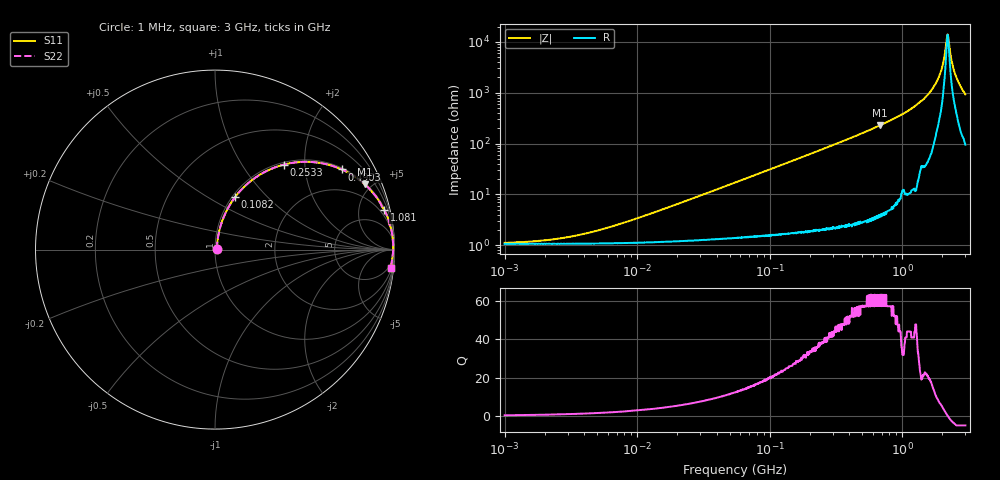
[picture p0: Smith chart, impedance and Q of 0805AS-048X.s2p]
!s-Parameter Generated by FASTRON Sdn. Bhd.
!FASTRON P/N : 0805AS-048X
!Keysight Technologies: E4991B_MY54100416_A.01.15
!Date: Mon Jun 15 12:50:52 2026
!Version  :Rev01  Mon Jun 15 12:50:52 2026
!Data & Calibration Information:
!Freq  S11  S21  S12  S22
!PortZ  Port1:50+j0  Port2:50+j0
!When reading reference impedance value at option line is always used.
! Remarks : This data is being provided solely for informational purposes.
# Hz S dB R 50
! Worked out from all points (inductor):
!   1601 points, 1 MHz to 3 GHz, reference 50 ohm
!   read as one part in series: L = 50.4 nH near 10.56 MHz
!   highest Q = 63.2 at 682.1 MHz (marker M1), where L = 53.2 nH
!   self-resonance near 2.2 GHz
!   S11 on the Smith chart (normalised r, x): 1 MHz: 1.02, +0.01; 108.2 MHz: 1.03, +0.67; 253.3 MHz: 1.04, +1.57; 490.3 MHz: 1.06, +3.13; 1.081 GHz: 1.20, +8.47; 3 GHz: 3, -19
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1000000  -39.20 16.7  -0.09 -0.2  -0.09 -0.2  -39.20 16.7
3804036  -35.90 48.2  -0.09 -0.7  -0.09 -0.7  -35.90 48.2
1.447069e7  -26.60 73.3  -0.11 -2.6  -0.11 -2.6  -26.60 73.3
5.504702e7  -15.60 75.8  -0.24 -9.5  -0.24 -9.5  -15.60 75.8
1.081723e8  -10.10 69.1  -0.58 -18.1  -0.58 -18.1  -10.10 69.1
2.083556e8  -5.47 56.1  -1.61 -32.2  -1.61 -32.2  -5.47 56.1
2.532562e8  -4.31 51.0  -2.18 -37.5  -2.18 -37.5  -4.31 51.0
4.902556e8  -1.56 32.3  -5.44 -56.7  -5.44 -56.7  -1.56 32.3
6.821091e8  -0.82 23.5  -7.97 -65.5  -7.97 -65.5  -0.82 23.5
7.925923e8  -0.59 19.9  -9.36 -69.1  -9.36 -69.1  -0.59 19.9
1.080907e9  -0.28 13.2  -12.80 -75.4  -12.80 -75.4  -0.28 13.2
1.474099e9  -0.12 7.3  -17.90 -80.1  -17.90 -80.1  -0.12 7.3
1.76507e9  -0.07 4.0  -23.20 -81.2  -23.20 -81.2  -0.07 4.0
1.970482e9  -0.06 2.1  -28.70 -78.0  -28.70 -78.0  -0.06 2.1
2.050964e9  -0.06 1.3  -32.40 -73.3  -32.40 -73.3  -0.06 1.3
2.145442e9  -0.06 0.5  -39.10 -51.9  -39.10 -51.9  -0.06 0.5
2.199798e9  -0.06 0.0  -43.00 -6.3  -43.00 -6.3  -0.06 0.0
2.255531e9  -0.07 -0.4  -39.70 43.8  -39.70 43.8  -0.07 -0.4
2.39512e9  -0.08 -1.5  -31.10 70.7  -31.10 70.7  -0.08 -1.5
2.51802e9  -0.09 -2.4  -27.20 74.9  -27.20 74.9  -0.09 -2.4
2.75535e9  -0.11 -4.2  -22.60 78.2  -22.60 78.2  -0.11 -4.2
3e9  -0.14 -6.0  -19.50 78.1  -19.50 78.1  -0.14 -6.0
